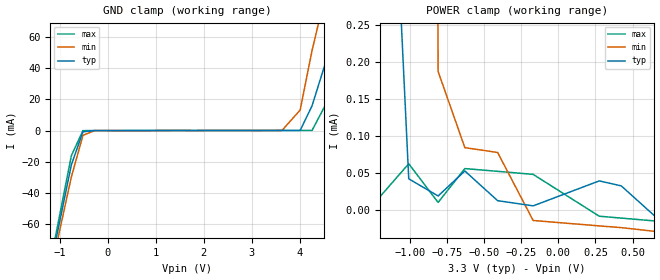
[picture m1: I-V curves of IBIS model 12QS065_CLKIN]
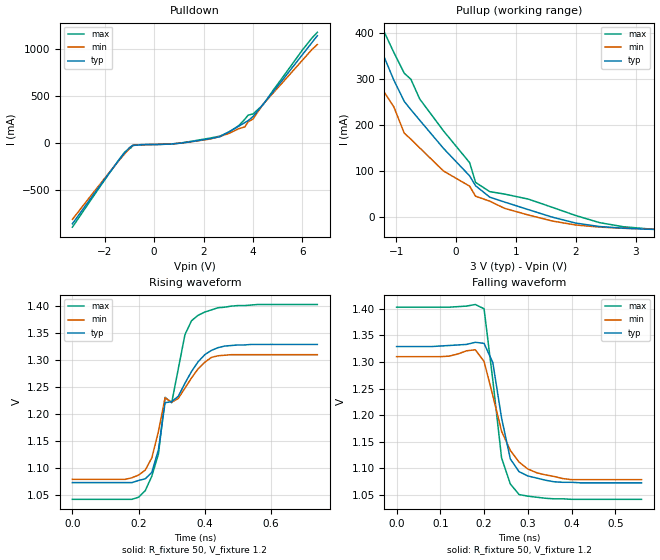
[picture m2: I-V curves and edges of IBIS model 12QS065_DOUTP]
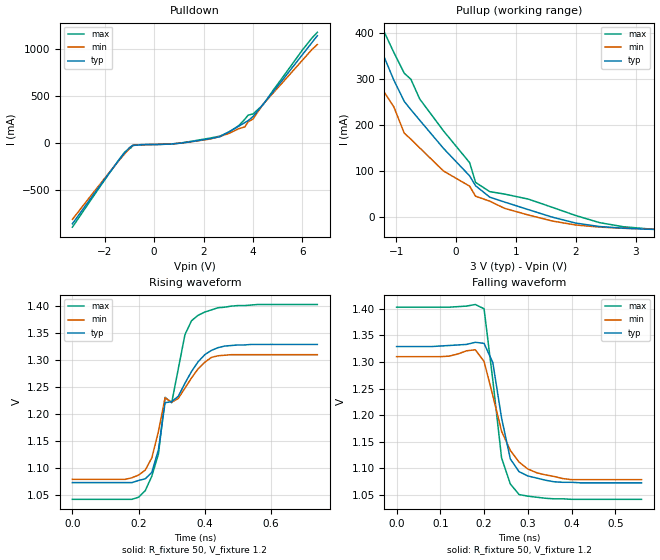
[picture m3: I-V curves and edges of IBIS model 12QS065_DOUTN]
|   National Semiconductor Corporation
|   Data Conversion Products Group
|   IBIS Model of ADC12QS065
|   60 Lead LLP Package
[IBIS Ver]   3.2
[File name]   adc12qs065.ibs
[File Rev]   1.2
[Date]   08/22/2006
[Source]   Bench Test to Ibis Conversion.
[Notes]   File created by RC,RL,IK.
Warnings: The CLKIN pin Power Clamp, and Ground Clamp Data is non-monotonic
   The MIN Column for the Rising and Falling Waveforms matches the
   calculated I/V curves with only 5% Accuracy. A more accurate MIN table
   may be provided at a later date.
[Disclaimer]
(C) Copyright National Semiconductor Corporation 2006
   All rights reserved
   National Semiconductor Corporation hereby grants
the user of this IBIS model a non-exclusive, nontransferable
license to use this IBIS model under the following terms.
Before using this IBIS model, the user should read this
license.  If the user does not accept these terms,  the
IBIS model should be returned to National within 30 days.
   The user is granted this license only to use the
IBIS model and is not granted rights to sell, load, rent,
lease or license the IBIS model in whole or in part, or in
modified form to anyone other than user. User may modify
the IBIS model to suit its specific applications but rights
to derivative works and such modifications shall belong to
National.
   This IBIS model is provided on an "AS IS" basis and
National makes absolutely no warranty with respect to the
information contained herein.NATIONAL DISCLAIMS AND CUSTOMER
WAIVES ALL WARRANTIES, EXPRESS OR IMPLIED, INCLUDING
WARRANTIES OF MERCHANTABILITY OR FITNESS FOR A PARTICULAR
PURPOSE. The entire risk as to quality and performance is
with the Customer. ACCORDINGLY, IN NO EVENT SHALL THE
COMPANY BE LIABLE FOR ANY DAMAGES, WHETHER IN CONTRACT OR
TORT,INCLUDING ANY LOST PROFITS OR OTHER INCIDENTAL,
CONSEQUENTIAL, EXEMPLARY, OR PUNITIVE DAMAGES ARISING OUT
OF THE USE OR APPLICATION OF THE IBIS model provided in
this package.Further, National reserves the right to make
changes without notice to any product herein to improve
reliability, function, or design. National does not convey
any license under patent rights or any other intellectual
property rights, including those of third parties.
   National is not obligated to provide maintenance or support
for the licensed IBIS model.
Contact National at ATTN:DCS APPLICATIONS/IBIS MODELS.
2900 Semiconductor Drive, M/S D3-739, Santa Clara, CA 95052-8090
[Copyright]   Copyright 2006, National Semiconductor, All Rights Reserved
[Component]   ADC12QS065
[Manufacturer]  National Semiconductor Corp
[Package]
|   typ   min   max
R_pkg   0.312   0.122   0.478
L_pkg   1.620nH   0.713nH   2.152nH
C_pkg   0.039pF   0.033pF   0.054pF
[Pin]   signal_name   model_name   R_pin   L_pin   C_pin
1   VA   POWER   0.023   1.610n   0.052p
2   AGND   GND   0.423   2.053n   0.036p
3   VIN1+   NC
4   VIN1-   NC
5   AGND   GND   0.196   1.280n   0.0036p
6   VIN2-   NC
7   VIN2+   NC
8   AGND   GND   0.368   1.804n   0.037p
9   VIN3+   NC
10   VIN3-   NC
11   AGND   GND   0.196   1.300n   0.036p
12   VIN4-   NC
13   VIN4+   NC
14   AGND   GND   0.226   1.520n   0.038p
15   VA   POWER   0.231   1.597n   0.057p
16   AGND   GND   0.430   2.173n   0.057p
17   VA   POWER   0.390   1.940n   0.036p
18   AGND   GND   0.351   1.710n   0.039p
19   VA   POWER   0.317   1.535n   0.035p
20   VREFB34   NC
21   VREFT34   NC
22   VCOM34   NC
23   VREF   NC
24   PD   NC
25   REFPD   NC
26   VD   POWER   0.190   1.216n   0.036p
27   DGND   GND   0.215   1.329n   0.035p
28   VDR   POWER   0.225   0.713n   0.039p
29   VREG   NC
30   DRGND   GND   0.239   2.394n   0.057p
31   DO4+   12QS065_DOUTP   0.478   2.208n   0.055p
32   D04-   12QS065_DOUTN   0.444   2.103n   0.036p
33   D03+   12QS065_DOUTP   0.423   1.951n   0.039p
34   D03-   12QS065_DOUTN   0.396   1.412n   0.036p
35   DRGND   GND   0.204   1.855n   0.036p
36   OUTCLK+   12QS065_DOUTP   0.379   1.805n   0.034p
37   OUTCLK-   12QS065_DOUTN   0.368   1.819n   0.038p
38   FRAME+   12QS065_DOUTP   0.370   1.794n   0.036p
39   FRAME-   12QS065_DOUTN   0.366   1.334n   0.038p
40   DRGND   GND   0.195   1.818n   0.035p
41   DO2+   12QS065_DOUTP   0.372   1.897n   0.035p
42   DO2-   12QS065_DOUTN   0.385   2.012n   0.035p
43   DO1+   12QS065_DOUTP   0.407   2.134n   0.039p
44   DO1-   12QS065_DOUTN   0.433   1.640n   0.038p
45   DRGND   GND   0.233   2.203n   0.055p
46   AGND   GND   0.436   1.935n   0.056p
47   CLK   12QS065_CLKIN   0.393   1.673n   0.037p
48   CLKB   GND   0.342   1.482n   0.039p
49   AGND   GND   0.305   1.352n   0.035p
50   DRGND   GND   0.283   1.236n   0.033p
51   VDR   POWER   0.274   0.904n   0.038p
52   DGND   GND   0.145   0.910n   0.038p
53   VD   POWER   0.141   1.282n   0.036p
54   INTREF   NC
55   VCOM12   NC
56   VREFT12   NC
57   VREFB12   NC
58   VA   POWER   0.376   1.663n   0.039p
59   VA   POWER   0.407   1.847n   0.037p
60   AGND   GND   0.434   2.152n   0.054p
[Diff_pin]   inv_pin   vdiff   tdelay_typ   tdelay_min   tdelay_max
| The '+' pin is Diff_pin and the '-' pin is the inv_pin
31   32   NA   0   0   0
33   34   NA   0   0   0
36   37   NA   0   0   0
38   39   NA   0   0   0
41   42   NA   0   0   0
43   44   NA   0   0   0
| Models and submodels in the file (3): 12QS065_CLKIN (Input), 12QS065_DOUTP (Output), 12QS065_DOUTN (Output)
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|   Clock Input MODEL
[Model]   12QS065_CLKIN
Model_type Input
Vinh=2.0
Vinl=0.8
|   TYP   MIN   MAX
C_comp   0.1p   0.1p   0.1p
[Temperature Range] 25   90   -20
[Voltage Range]   3.3   3.0   3.6
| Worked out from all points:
|   GND clamp passes 1 mA (typ) near -0.52 V on its own axis
|   POWER clamp passes 1 mA (typ) near -1.21 V on its own axis
[GND Clamp]
|V(groundclamp)   I(typ)   I(min)   I(max)
-3V       -376mA     -362mA     -388mA
-1.157V   -81.1mA    -85.4mA    -78mA
-760.6mV  -22mA      -29.7mA    -16.1mA
-519.1mV  -806uA     -3.11mA    -72uA
-277.5mV  -52.7uA    -12.9uA    -10.5uA
3.63V     53uA       84.4uA     56.2uA
4.008V    42.4uA     13.1mA     62.7uA
4.256V    15.8mA     51.1mA     67uA
4.726V    61.9mA     112mA      27.4mA
5.182V    164mA      211mA      109mA
5.974V    306mA      344mA      257mA
[POWER Clamp]
|V(table)   I(typ)   I(min)   I(max)
-3.172V   341mA      378mA      295mA
-1.503V   40.2mA     80.3mA     774uA
-1.256V   15.8mA     51.1mA     67uA
-1.206V   875uA      30.3mA     17.4uA
-1.008V   42.4uA     13.1mA     62.7uA
-810.2mV  19.3uA     187uA      10.6uA
-630mV    53uA       84.4uA     56.2uA
-409.3mV  13uA       77.9uA     52.5uA
-169.7mV  5.99uA     -13.7uA    48.4uA
275.8mV   39.6uA     -21uA      -7.95uA
424.3mV   32.9uA     -23.3uA    -10.5uA
643.1mV   -6.48uA    -28.2uA    -14.2uA
|   Driver Output MODELs
[Model]   12QS065_DOUTP
Model_type Output
Polarity Non-Inverting
Vref=1.2
Vmeas=1.2
Rref=50
Cref=5p
|   TYP   MIN   MAX
C_comp   0.1p   0.1p   0.1p
[Temperature Range] 25   90   -20
[Voltage Range]   3.0   2.7   3.6
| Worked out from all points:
|   slope of the pulldown table from 0 to 0.45 V, typ, clamps not added: 171 ohm
|   slope of the pullup table from 0 to 0.45 V, typ, clamps not added: 6.9 ohm
|   falling waveform, R_fixture 50, V_fixture 1.2: 20-80 % time 34.3ps typ, 56.4ps min, 32ps max; typ from 1.33 V to 1.07 V
|   rising waveform, R_fixture 50, V_fixture 1.2: 20-80 % time 104ps typ, 114ps min, 80.6ps max; typ from 1.07 V to 1.33 V
[Pullup]
|Vtable   I(typ)   I(min)   I(max)
-5.776V   1.872A     1.608A     2.067A
-2.014V   613mA      496mA      698mA
-1.618V   482mA      381mA      555mA
-1.222V   353mA      275mA      407mA
-1.041V   297mA      239mA      357mA
-867.9mV  251mA      182mA      312mA
-212.5mV  149mA      100mA      187mA
224.4mV   89.4mA     67mA       118mA
324.1mV   67.9mA     45.2mA     75.2mA
559.7mV   43.3mA     34.5mA     55.2mA
1.995V    -13mA      -17.2mA    3.42mA
3.3V      -26.8mA    -26.5mA    -26.6mA
[Pulldown]
|V(pulldown)   I(typ)   I(min)   I(max)
-3.3V     -854mA     -808mA     -890mA
-1.427V   -180mA     -185mA     -177mA
-884.4mV  -26.6mA    -28.3mA    -23.1mA
1.479V    17.2mA     16.3mA     20.8mA
2.659V    70.7mA     72.8mA     76.7mA
3.027V    122mA      106mA      121mA
3.671V    221mA      175mA      257mA
3.804V    241mA      229mA      300mA
4.002V    286mA      260mA      313mA
4.408V    415mA      416mA      410mA
5.992V    941mA      882mA      990mA
6.6V      1.144A     1.05A      1.18A
[Ramp]
|   TYP   MIN   MAX
dV/dt_r   0.144/95.1E-12   0.144/121.2e-12   0.144/79.23e-12
dV/dt_f   0.195/27.9e-12   0.195/34.02e-12   0.195/22.35e-12
R_load=50
[Falling Waveform]
R_fixture=50
V_fixture=1.2
| 100 Ohms Across Outputs DOUTP and DOUTN
|Time   V(typ)   V(min)   V(max)
0s        1.329V     1.31V      1.403V
120ps     1.331V     1.311V     1.403V
180ps     1.337V     1.323V     1.408V
200ps     1.335V     1.301V     1.4V
220ps     1.299V     1.237V     1.266V
240ps     1.195V     1.17V      1.12V
260ps     1.118V     1.134V     1.071V
280ps     1.094V     1.112V     1.051V
380ps     1.074V     1.081V     1.043V
560ps     1.073V     1.079V     1.042V
[Rising Waveform]
R_fixture=50
V_fixture=1.2
|Time   V(typ)   V(min)   V(max)
0s        1.073V     1.079V     1.042V
220ps     1.08V      1.096V     1.058V
240ps     1.092V     1.119V     1.085V
260ps     1.134V     1.168V     1.126V
280ps     1.221V     1.23V      1.231V
300ps     1.223V     1.222V     1.221V
340ps     1.257V     1.248V     1.347V
380ps     1.297V     1.284V     1.383V
460ps     1.326V     1.309V     1.398V
740ps     1.329V     1.31V      1.403V
[Model]   12QS065_DOUTN
Model_type Output
Polarity Inverting
Vref=1.2
Vmeas=1.2
Rref=50
Cref=5p
|   TYP   MIN   MAX
C_comp   0.1p   0.1p   0.1p
[Temperature Range] 25   90   -20
[Voltage Range]   3.0   2.7   3.6
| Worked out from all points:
|   slope of the pulldown table from 0 to 0.45 V, typ, clamps not added: 171 ohm
|   slope of the pullup table from 0 to 0.45 V, typ, clamps not added: 6.9 ohm
|   falling waveform, R_fixture 50, V_fixture 1.2: 20-80 % time 34.3ps typ, 56.4ps min, 32ps max; typ from 1.33 V to 1.07 V
|   rising waveform, R_fixture 50, V_fixture 1.2: 20-80 % time 104ps typ, 114ps min, 80.6ps max; typ from 1.07 V to 1.33 V
[Pullup]
|Vtable   I(typ)   I(min)   I(max)
-5.776V   1.872A     1.608A     2.067A
-2.014V   613mA      496mA      698mA
-1.618V   482mA      381mA      555mA
-1.222V   353mA      275mA      407mA
-1.041V   297mA      239mA      357mA
-867.9mV  251mA      182mA      312mA
-212.5mV  149mA      100mA      187mA
224.4mV   89.4mA     67mA       118mA
324.1mV   67.9mA     45.2mA     75.2mA
559.7mV   43.3mA     34.5mA     55.2mA
1.995V    -13mA      -17.2mA    3.42mA
3.3V      -26.8mA    -26.5mA    -26.6mA
[Pulldown]
|V(pulldown)   I(typ)   I(min)   I(max)
-3.3V     -854mA     -808mA     -890mA
-1.427V   -180mA     -185mA     -177mA
-884.4mV  -26.6mA    -28.3mA    -23.1mA
1.479V    17.2mA     16.3mA     20.8mA
2.659V    70.7mA     72.8mA     76.7mA
3.027V    122mA      106mA      121mA
3.671V    221mA      175mA      257mA
3.804V    241mA      229mA      300mA
4.002V    286mA      260mA      313mA
4.408V    415mA      416mA      410mA
5.992V    941mA      882mA      990mA
6.6V      1.144A     1.05A      1.18A
[Ramp]
|   TYP   MIN   MAX
dV/dt_r   0.144/95.1E-12   0.144/121.2e-12   0.144/79.23e-12
dV/dt_f   0.195/27.9e-12   0.195/34.02e-12   0.195/22.35e-12
R_load=50
[Falling Waveform]
R_fixture=50
V_fixture=1.2
| 100 Ohms Across Outputs DOUTP and DOUTN
|Time   V(typ)   V(min)   V(max)
0s        1.329V     1.31V      1.403V
120ps     1.331V     1.311V     1.403V
180ps     1.337V     1.323V     1.408V
200ps     1.335V     1.301V     1.4V
220ps     1.299V     1.237V     1.266V
240ps     1.195V     1.17V      1.12V
260ps     1.118V     1.134V     1.071V
280ps     1.094V     1.112V     1.051V
380ps     1.074V     1.081V     1.043V
560ps     1.073V     1.079V     1.042V
[Rising Waveform]
R_fixture=50
V_fixture=1.2
|Time   V(typ)   V(min)   V(max)
0s        1.073V     1.079V     1.042V
220ps     1.08V      1.096V     1.058V
240ps     1.092V     1.119V     1.085V
260ps     1.134V     1.168V     1.126V
280ps     1.221V     1.23V      1.231V
300ps     1.223V     1.222V     1.221V
340ps     1.257V     1.248V     1.347V
380ps     1.297V     1.284V     1.383V
460ps     1.326V     1.309V     1.398V
740ps     1.329V     1.31V      1.403V
